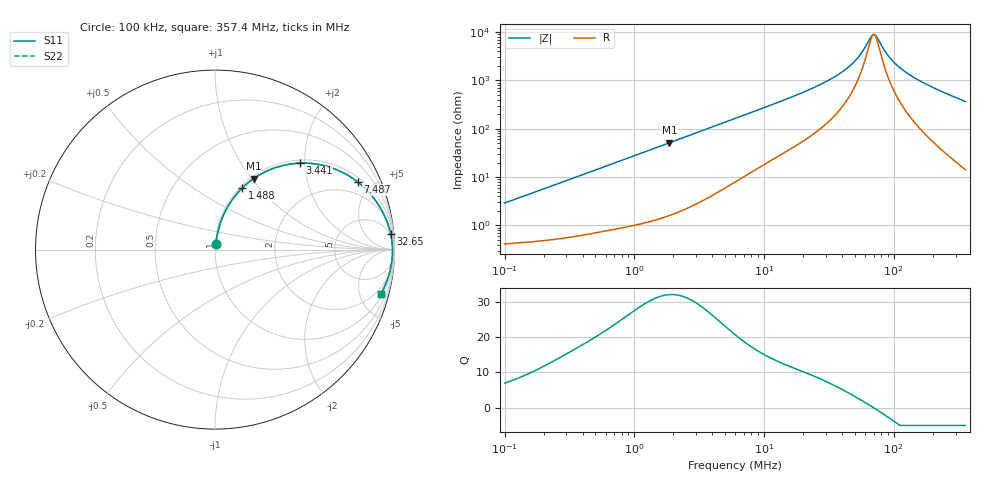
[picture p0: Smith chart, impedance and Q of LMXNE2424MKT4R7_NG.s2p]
! LMXNE2424MKT4R7_NG  S-PARAMETER MODEL  ( General Type )
! Model Generated by TAIYO YUDEN Corporation (https://www.yuden.co.jp/en/)
! Version 1.0
! TAIYO YUDEN Control No. 191023NI43SB-FBB
! Copyright(c) 2019 TAIYO YUDEN CO.,LTD. All Rights Reserved.
! Product Description (link to TY-COMPAS)
! https://ds.yuden.co.jp/TYCOMPAS/or/detail?pn=LMXNE2424MKT4R7MNG&u=M
! Products Name : Inductors
! Characteristics :
!  Inductance : 4.7 uH , SRF(min) : 45 MHz , DC Resistance(max) : 0.36 Ohm
!  Rated Current : Saturation :1150 mA , Temp Rise : 650 mA (40 degC)
!  Case Size : 2.4 x 2.4 / 0.095 x 0.095 [mm/inch] , Thickness : 1.2 / 0.047 [mm/inch]
!  (Conditions: Temperature = 25 degC , DC Bias Current/Voltage = 0A / 0V)
! External Node Assignments :
!  1  o---GGG---o  2
! GND o---------o GND
! Frequency Range : 0.1MHz  -  357.398349MHz  [ 402 STEP ]
# MHz S RI R 50
! Freq[MHz].  S11 Real  S11 Imag  S21 Real  S21 Imag  S12 Real  S12 Imag  S22 Real  S22 Imag
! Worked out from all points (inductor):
!   401 points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, 100 kHz to 357.4 MHz, reference 50 ohm
!   read as one part in series: L = 4.55 uH near 104.2 kHz
!   highest Q = 32.1 at 1.863 MHz (marker M1), where L = 4.37 uH
!   self-resonance near 69.59 MHz
!   S11 on the Smith chart (normalised r, x): 100 kHz: 1.01, +0.06; 1.488 MHz: 1.03, +0.82; 3.441 MHz: 1.07, +1.89; 7.487 MHz: 1.23, +4.08; 32.65 MHz: 4, +21; 357.4 MHz: 1.29, -7.34
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0.1  0.00493 0.0285  0.9951 -0.0285  0.9951 -0.0285  0.00493 0.0285
0.393689  0.018 0.1077  0.982 -0.1077  0.982 -0.1077  0.018 0.1077
0.856451  0.0609 0.2205  0.9391 -0.2205  0.9391 -0.2205  0.0609 0.2205
1.487786  0.1515 0.3428  0.8485 -0.3428  0.8485 -0.3428  0.1515 0.3428
1.549909  0.1617 0.3526  0.8383 -0.3526  0.8383 -0.3526  0.1617 0.3526
1.863168  0.215 0.3955  0.785 -0.3955  0.785 -0.3955  0.215 0.3955
3.441426  0.4718 0.4818  0.5282 -0.4818  0.5282 -0.4818  0.4718 0.4818
6.101817  0.7259 0.4223  0.2741 -0.4223  0.2741 -0.4223  0.7259 0.4223
7.486658  0.7941 0.3775  0.2059 -0.3775  0.2059 -0.3775  0.7941 0.3775
12.48418  0.9051 0.2579  0.0949 -0.2579  0.0949 -0.2579  0.9051 0.2579
23.53582  0.965 0.1373  0.035 -0.1373  0.035 -0.1373  0.965 0.1373
32.64791  0.9784 0.0895  0.0216 -0.0895  0.0216 -0.0895  0.9784 0.0895
40.88529  0.9839 0.0609  0.0161 -0.0609  0.0161 -0.0609  0.9839 0.0609
49.14881  0.9867 0.0394  0.0133 -0.0394  0.0133 -0.0394  0.9867 0.0394
55.56615  0.9879 0.0256  0.0121 -0.0256  0.0121 -0.0256  0.9879 0.0256
65.44454  0.9888 0.00769  0.0112 -0.00769  0.0112 -0.00769  0.9888 0.00769
69.58603  0.989 0.00103  0.011 -0.00103  0.011 -0.00103  0.989 0.00103
73.9896  0.9891 -0.00563  0.0109 0.00563  0.0109 0.00563  0.9891 -0.00563
92.65788  0.9884 -0.0304  0.0116 0.0304  0.0116 0.0304  0.9884 -0.0304
113.6871  0.9865 -0.0542  0.0135 0.0542  0.0135 0.0542  0.9865 -0.0542
151.3811  0.9811 -0.0912  0.0189 0.0912  0.0189 0.0912  0.9811 -0.0912
357.3983  0.9227 -0.2483  0.0773 0.2483  0.0773 0.2483  0.9227 -0.2483
